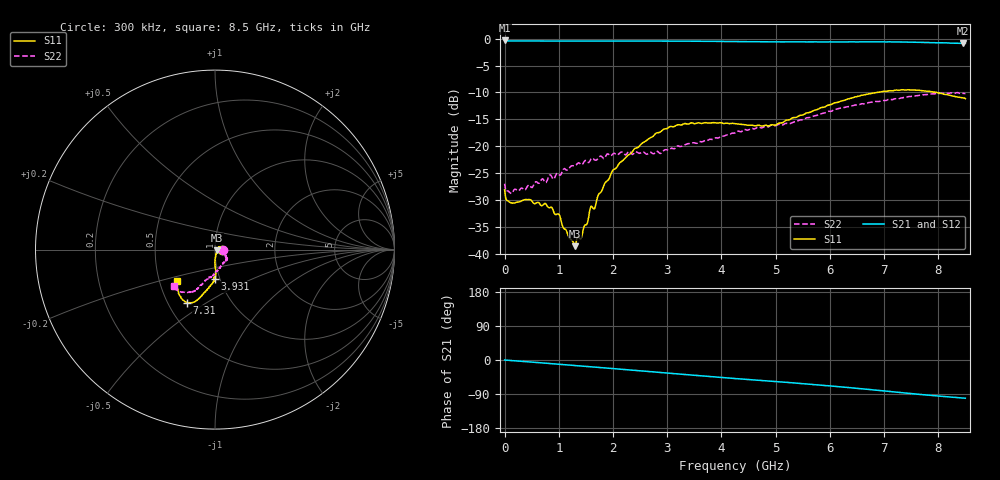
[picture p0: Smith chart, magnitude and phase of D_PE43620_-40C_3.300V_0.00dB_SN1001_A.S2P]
! device id: pe43620
! dir: c:\dsa\pe43620\data\pe43620\-40c\3p300v\00p00db
! Serial: 1001
! Insertion: A
! Temp: -40C
! VDD: 3.300V
! Attenuation Step: 0.00dB
! IDD: 8.563861e-03mA
! FILE NAME
! DATE 10-22-2008 14:40:12
! CORRECTED  DATA
#  Hz  S  RI  R  50.00
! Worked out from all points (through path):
!   401 points, 300 kHz to 8.5 GHz, reference 50 ohm
!   highest |S21| = -0.33 dB at 300 kHz (marker M1); lowest = -0.9 dB at 8.458 GHz (marker M2)
!   group delay of S21, straight-line fit = 32.8 ps
!   lowest |S11| = -38.6 dB at 1.297 GHz (marker M3), VSWR 1.02, Z = 51.1 - j0.351 ohm
!   |S11| at or under -10 dB: start of sweep to 6.872 GHz; 7.971 GHz to end of sweep
!   |S22| runs from -28.8 to -10.0 dB; largest |S21 - S12| = 0.0053
!   S11 on the Smith chart (normalised r, x): 300 kHz: 1.08, +0.00; 3.931 GHz: 0.95, -0.32; 7.31 GHz: 0.62, -0.42; 8.5 GHz: 0.61, -0.24
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300000  0.0393 0.00025  0.9625 -0.00124  0.9628 -8.51e-05  0.0447 -0.00123
1.277955e8  0.0296 0.00235  0.9526 -0.0248  0.9529 -0.0254  0.0361 -0.00407
4.465343e8  0.0284 0.0146  0.9484 -0.0818  0.9488 -0.0818  0.043 -0.00703
8.5027e8  0.0227 0.0147  0.9386 -0.1552  0.9395 -0.1558  0.0506 -0.0191
9.990148e8  0.0201 0.0119  0.9334 -0.1824  0.9339 -0.1832  0.0501 -0.022
1.211507e9  0.0136 -0.0017  0.9243 -0.2222  0.9252 -0.2222  0.0569 -0.0305
1.296504e9  0.0113 -0.00343  0.9208 -0.2375  0.9207 -0.2378  0.0569 -0.0326
1.424e9  0.00957 -0.0107  0.9141 -0.2616  0.9145 -0.2615  0.0581 -0.0338
1.593994e9  0.00691 -0.0268  0.9043 -0.2917  0.905 -0.2925  0.0633 -0.042
1.99773e9  0.000181 -0.0599  0.8768 -0.3652  0.8788 -0.3645  0.0666 -0.0523
2.401465e9  0.00122 -0.0952  0.8433 -0.4364  0.8441 -0.4369  0.0633 -0.0607
2.8477e9  0.00646 -0.1338  0.8001 -0.5114  0.8011 -0.5113  0.0453 -0.0743
3.315183e9  -0.000561 -0.1622  0.746 -0.5851  0.7467 -0.5854  0.03 -0.0977
3.931411e9  0.00059 -0.1642  0.666 -0.6696  0.6657 -0.6708  0.00779 -0.1189
4.25015e9  -0.00276 -0.1619  0.6196 -0.7088  0.6191 -0.7089  -0.0028 -0.1329
4.972625e9  -0.000468 -0.1569  0.5135 -0.7789  0.5107 -0.78  -0.0262 -0.1531
5.67385e9  -0.0335 -0.2092  0.4007 -0.8419  0.4017 -0.8435  -0.0604 -0.1784
6.481321e9  -0.0902 -0.2737  0.2485 -0.9002  0.2516 -0.9009  -0.0993 -0.2207
7.09755e9  -0.138 -0.2978  0.1148 -0.9284  0.1125 -0.9279  -0.1318 -0.2401
7.310042e9  -0.1563 -0.2957  0.0671 -0.9292  0.0643 -0.9301  -0.1493 -0.2381
8.457502e9  -0.2158 -0.182  -0.1647 -0.8884  -0.1644 -0.8906  -0.2316 -0.2066
8.5e9  -0.2135 -0.1767  -0.1715 -0.8875  -0.1737 -0.8881  -0.2303 -0.2041
